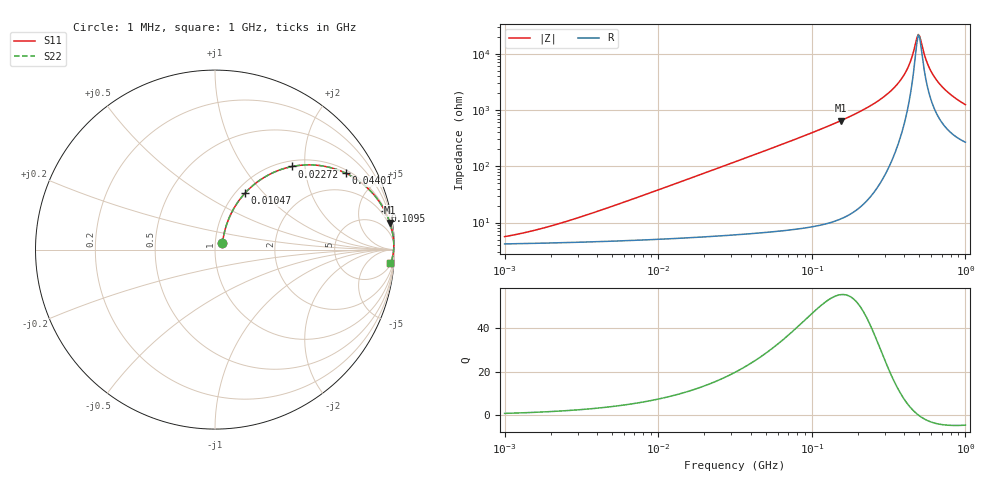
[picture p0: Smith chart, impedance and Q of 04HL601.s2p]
! Coilcraft 0402HL-601 Chip Inductor
! 2 August 2012
# MHz S MA R 50
!Freq  MagS11  AngS11  MagS21  AngS21  MagS12  AngS12  MagS22  AngS22
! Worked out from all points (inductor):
!   304 points, 1 MHz to 1 GHz, reference 50 ohm
!   read as one part in series: L = 600 nH near 3.667 MHz
!   highest Q = 55.5 at 154.2 MHz (marker M1), where L = 664 nH
!   self-resonance near 493.3 MHz
!   S11 on the Smith chart (normalised r, x): 1 MHz: 1.08, +0.08; 10.47 MHz: 1.10, +0.79; 22.72 MHz: 1.11, +1.72; 44.01 MHz: 1.13, +3.34; 109.5 MHz: 1.18, +8.68; 1 GHz: 6, -24
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1  0.054 40.0  0.9592 -2.1  0.9592 -2.1  0.054 40.0
3.19853  0.1223 63.0  0.9507 -6.6  0.9507 -6.6  0.1223 63.0
10  0.3409 62.6  0.896 -19.7  0.896 -19.7  0.3409 62.6
10.46651  0.3546 62.1  0.8909 -20.6  0.8909 -20.6  0.3546 62.1
22.72143  0.6318 47.1  0.7344 -39.1  0.7344 -39.1  0.6318 47.1
31.9853  0.7532 38.3  0.6212 -48.8  0.6212 -48.8  0.7532 38.3
44.01132  0.8442 30.3  0.5044 -57.5  0.5044 -57.5  0.8442 30.3
102.306  0.9658 13.9  0.2397 -74.9  0.2397 -74.9  0.9658 13.9
109.5479  0.9702 12.9  0.2234 -75.9  0.2234 -75.9  0.9702 12.9
154.2122  0.9855 8.8  0.1531 -80.2  0.1531 -80.2  0.9855 8.8
237.8141  0.9943 4.9  0.0854 -83.7  0.0854 -83.7  0.9943 4.9
319.853  0.9965 2.8  0.04833 -84.4  0.04833 -84.4  0.9965 2.8
375.1953  0.9967 1.7  0.03033 -82.8  0.03033 -82.8  0.9967 1.7
420.4965  0.9964 1.0  0.0181 -78.1  0.0181 -78.1  0.9964 1.0
450.2621  0.9961 0.6  0.01114 -69.4  0.01114 -69.4  0.9961 0.6
493.2525  0.9955 0.0  0.004543 -10.2  0.004543 -10.2  0.9955 0.0
504.6268  0.9953 -0.1  0.004925 18.9  0.004925 18.9  0.9953 -0.1
540.3477  0.9947 -0.5  0.01027 58.6  0.01027 58.6  0.9947 -0.5
565.5555  0.9942 -0.8  0.01478 66.4  0.01478 66.4  0.9942 -0.8
633.8408  0.9926 -1.5  0.02669 73.1  0.02669 73.1  0.9926 -1.5
760.6557  0.9889 -2.6  0.04666 74.9  0.04666 74.9  0.9889 -2.6
1000  0.98 -4.4  0.07896 73.1  0.07896 73.1  0.98 -4.4
